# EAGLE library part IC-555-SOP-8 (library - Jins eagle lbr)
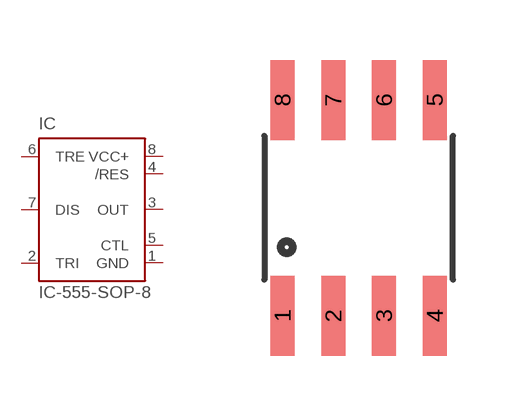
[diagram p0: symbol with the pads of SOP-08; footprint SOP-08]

Designator prefix IC

## IC-555-SOP-8  [SOP-08]
1  GND  pwr
2  TRI  in
3  OUT  out
4  /RES  in
5  CTL  in
6  TRE  in
7  DIS  in
8  VCC+  pwr

## Footprint SOP-08 (pad centres in mm)
smd 0.6 x 2: 1 -1.905,-2.7; 2 -0.635,-2.7; 3 0.635,-2.7; 4 1.905,-2.7; 5 1.905,2.7; 6 0.635,2.7; 7 -0.635,2.7; 8 -1.905,2.7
